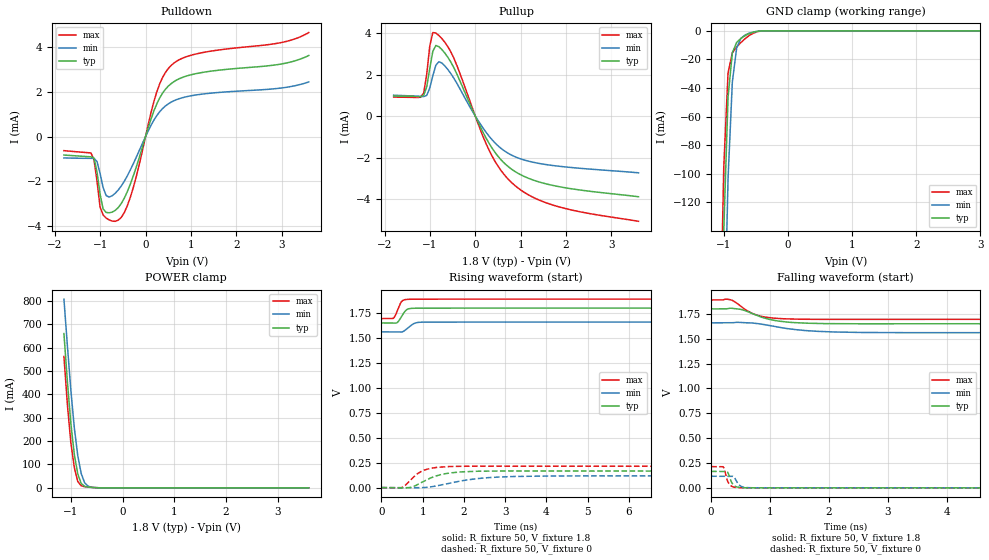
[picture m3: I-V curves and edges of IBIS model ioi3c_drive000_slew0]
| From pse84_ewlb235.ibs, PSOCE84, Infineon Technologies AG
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[Model] ioi3c_drive000_slew0
Model_type I/O
Enable   Active-High
Vinl  =  0.54
Vinh  =  1.26
Vmeas =  0.9
Cref  =  15e-12
| Capacitance   typ   min   max
C_comp   9.12545e-13 8.87504e-13 9.42456e-13
| Variables   typ   min   max
[GND Clamp Reference]   0   0   0
[POWER Clamp Reference]   1.8   1.66   1.89
[Pulldown Reference]   0   0   0
[Pullup Reference]   1.8   1.66   1.89
[Temperature Range]   25   125   -40
[Voltage Range]   1.8   1.66   1.89
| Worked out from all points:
|   slope of the pulldown table from 0 to 0.27 V, typ, clamps not added: 174 ohm
|   slope of the pullup table from 0 to 0.27 V, typ, clamps not added: 228 ohm
|   GND clamp passes 1 mA (typ) near -0.55 V on its own axis
|   POWER clamp passes 1 mA (typ) near -0.54 V on its own axis
|   falling waveform, R_fixture 50, V_fixture 1.8: 20-80 % time 483ps typ, 697ps min, 344ps max; typ from 1.8 V to 1.65 V
|   falling waveform, R_fixture 50, V_fixture 0: 20-80 % time 73.3ps typ, 80.7ps min, 69.2ps max; typ from 0.165 V to 0 V
|   rising waveform, R_fixture 50, V_fixture 1.8: 20-80 % time 140ps typ, 184ps min, 118ps max; typ from 1.65 V to 1.8 V
|   rising waveform, R_fixture 50, V_fixture 0: 20-80 % time 576ps typ, 998ps min, 388ps max; typ from 0 V to 0.165 V
[GND Clamp]
| Voltage   I(typ)   I(min)   I(max)
-1.204V   -737.9mA   -831.5mA   -678.7mA
-1.07V    -303.2mA   -410.8mA   -239.8mA
-1.003V   -139.9mA   -232.2mA   -95.74mA
-936.6mV  -46.51mA   -103.5mA   -29.5mA
-869.7mV  -15.31mA   -35.88mA   -15.36mA
-802.8mV  -8.166mA   -12.13mA   -11.29mA
-735.9mV  -5.335mA   -5.292mA   -8.195mA
-669mV    -3.356mA   -2.85mA    -5.457mA
-535.2mV  -837.9uA   -772uA     -1.483mA
-401.4mV  -47.36uA   -84.85uA   -76.77uA
3.6V      0A         0A         0A
[POWER Clamp]
| Voltage   I(typ)   I(min)   I(max)
-1.137V   660mA      807.5mA    561.8mA
-1.07V    454.5mA    608.2mA    356.2mA
-1.003V   275.7mA    418.4mA    193.6mA
-936.6mV  143.5mA    257.2mA    86.91mA
-869.7mV  59.43mA    137.9mA    27.31mA
-802.8mV  18.8mA     60.93mA    8.704mA
-735.9mV  6.231mA    21.35mA    5.155mA
-669mV    3.127mA    6.887mA    3.44mA
-535.2mV  940.9uA    1.232mA    1.058mA
-334.5mV  16.1uA     59.03uA    7.686uA
3.6V      0A         0A         0A
[Pulldown]
| Voltage   I(typ)   I(min)   I(max)
-1.8V     -827.2uA   -955.9uA   -630.1uA
-1.204V   -905.7uA   -974.4uA   -731.3uA
-1.137V   -966.5uA   -974.4uA   -1.034mA
-1.003V   -2.575mA   -1.645mA   -3.146mA
-936.6mV  -3.233mA   -2.275mA   -3.507mA
-802.8mV  -3.412mA   -2.706mA   -3.732mA
-602.1mV  -3.177mA   -2.391mA   -3.74mA
-267.6mV  -1.747mA   -1.204mA   -2.264mA
248.3mV   1.461mA    938uA      1.999mA
558.6mV   2.359mA    1.534mA    3.169mA
1.117V    2.817mA    1.863mA    3.696mA
3.6V      3.626mA    2.444mA    4.653mA
[Pullup]
| Voltage   I(typ)   I(min)   I(max)
-1.8V     968.9uA    1.007mA    914.8uA
-1.137V   998.9uA    941.3uA    1.117mA
-1.07V    1.412mA    996.9uA    2.02mA
-1.003V   2.299mA    1.357mA    3.386mA
-936.6mV  3.123mA    1.948mA    4.03mA
-869.7mV  3.405mA    2.453mA    4.01mA
-735.9mV  3.208mA    2.56mA     3.737mA
-468.3mV  2.317mA    1.812mA    2.775mA
310.3mV   -1.337mA   -986.1uA   -1.671mA
806.9mV   -2.573mA   -1.892mA   -3.221mA
1.738V    -3.359mA   -2.393mA   -4.312mA
3.6V      -3.894mA   -2.739mA   -5.079mA
[Ramp]
dV/dt_r   99.2904m/0.576369n  70.0417m/0.997596n  0.128112/0.388021n
dV/dt_f   89.3259m/0.482521n  58.9256m/0.697084n  0.116841/0.343645n
R_load = 50
[Falling Waveform]
R_fixture = 50
V_fixture = 1.8
V_fixture_min = 1.66
V_fixture_max = 1.89
| Time   V(typ)   V(min)   V(max)
0s        1.8V       1.66V      1.89V
258.5ps   1.8V       1.66V      1.898V
344.2ps   1.807V     1.66V      1.889V
521.4ps   1.793V     1.662V     1.819V
682ps     1.757V     1.659V     1.759V
933.2ps   1.703V     1.639V     1.716V
1.233ns   1.671V     1.607V     1.701V
1.821ns   1.654V     1.574V     1.695V
3.286ns   1.65V      1.561V     1.695V
800ns     1.651V     1.562V     1.695V
[Falling Waveform]
R_fixture = 50
V_fixture = 0
V_fixture_min = 0
V_fixture_max = 0
| Time   V(typ)   V(min)   V(max)
0s        165.5mV    116.7mV    213.5mV
204.6ps   165.4mV    116.7mV    210.7mV
264.4ps   164.9mV    116.7mV    92.33mV
289.2ps   147.2mV    116.6mV    54.66mV
341.8ps   61.67mV    117mV      18.29mV
381.5ps   27.64mV    111.2mV    7.842mV
469.8ps   5.125mV    32.14mV    1.422mV
542.6ps   1.606mV    8.122mV    649.2uV
1.139ns   229.6uV    339.5uV    140.1uV
800ns     22.46nV    1.283uV    9.56nV
[Rising Waveform]
R_fixture = 50
V_fixture = 1.8
V_fixture_min = 1.66
V_fixture_max = 1.89
| Time   V(typ)   V(min)   V(max)
0s        1.651V     1.562V     1.695V
290.8ps   1.651V     1.562V     1.699V
337.5ps   1.65V      1.562V     1.727V
395ps     1.66V      1.562V     1.782V
472ps     1.705V     1.56V      1.856V
545ps     1.753V     1.57V      1.882V
653ps     1.792V     1.606V     1.888V
856.8ps   1.799V     1.655V     1.889V
1.499ns   1.8V       1.66V      1.89V
800ns     1.8V       1.66V      1.89V
[Rising Waveform]
R_fixture = 50
V_fixture = 0
V_fixture_min = 0
V_fixture_max = 0
| Time   V(typ)   V(min)   V(max)
0s        22.46nV    1.283uV    9.56nV
492.9ps   -1.705mV   -160.2uV   572.4uV
720.1ps   3.928mV    -1.156mV   82.78mV
898ps     34.95mV    -878.6uV   146mV
1.193ns   96.54mV    7.482mV    193.4mV
1.517ns   137.1mV    32.36mV    208.3mV
2.089ns   160.1mV    77.58mV    214.9mV
3.264ns   166.8mV    112mV      214.5mV
4.973ns   166.1mV    117.6mV    213.7mV
50ns      165.5mV    116.7mV    213.5mV
